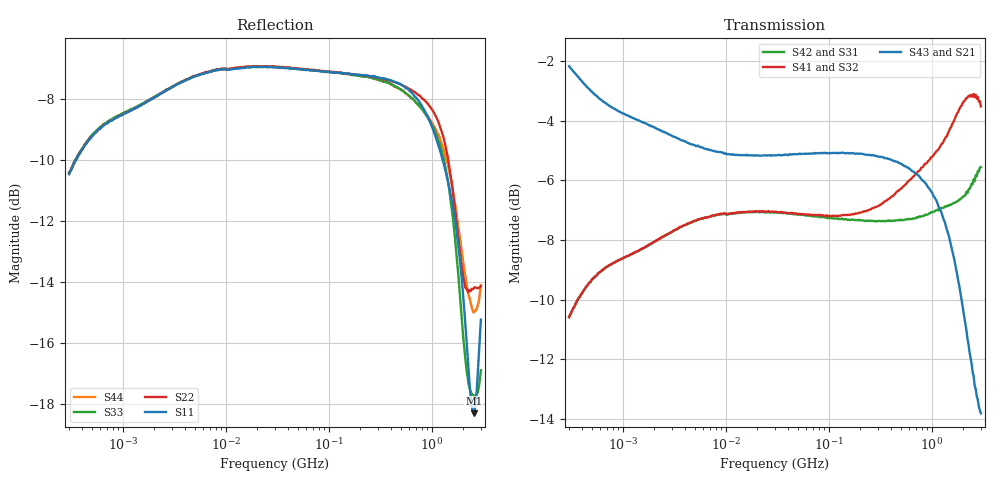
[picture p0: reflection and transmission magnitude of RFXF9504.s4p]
! RFMD Transformer
! RFXF9504 Tested 12/6/2010
! S4P Data File Format
! All S Parameters Mag in dB and Angle in Degree format
! Test Conditions: Input Power = -10dBm @ Temperature +25 deg C
! 401 Frequency points - Log Sweep
! Port 1 is Pin 1,Port 2 is Pin 4, Port 3 is Pin 3 and Port 4 is Pin 2
! FrequencMag(S11)Angle(S1Mag(S12)Angle(S1Mag(S13)Angle(S1Mag(S14)Angle(S14)
!  Mag(S21)Angle(S2Mag(S22)Angle(S2Mag(S23)Angle(S2Mag(S24)Angle(S24)
!  Mag(S31)Angle(S3Mag(S32)Angle(S3Mag(S33)Angle(S3Mag(S34)Angle(S34)
!  Mag(S41)Angle(S4Mag(S42)Angle(S4Mag(S43)Angle(S4Mag(S44)Angle(S44)
# Hz S  dB  R 50
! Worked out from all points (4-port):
!   401 points, 300 kHz to 3 GHz, reference 50 ohm
!   strongest paths, dB at 300 kHz, 3 MHz, 30 MHz, 300 MHz, 3 GHz:
!     S43: -2.2, -4.5, -5.2, -5.2, -13.8
!     S21: -2.2, -4.5, -5.2, -5.2, -14.5
!     S41: -10.6, -7.7, -7.0, -6.9, -3.5
!     S32: -10.6, -7.7, -7.1, -6.9, -3.5
!     S42: -10.6, -7.7, -7.1, -7.4, -5.5
!     S31: -10.6, -7.7, -7.1, -7.4, -5.3
!   lowest |S11| = -18.3 dB at 2.553 GHz (marker M1), VSWR 1.28, Z = 63.3 + j3.69 ohm
!   |S11| at or under -10 dB: start of sweep to 352.5 kHz; 1.274 GHz to end of sweep
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300000  -10.48 36.5  -2.18 -13.2  -10.54 -143.6  -10.54 -143.6
        -2.18 -13.1  -10.46 36.6  -10.53 36.5  -10.54 -143.3
        -10.58 -143.5  -10.56 36.6  -10.42 35.8  -2.17 -13.2
        -10.59 36.7  -10.58 -143.4  -2.17 -13.2  -10.43 36.1
386474.9  -9.76 30.7  -2.63 -12.9  -9.84 -149.3  -9.84 -149.3
          -2.63 -12.9  -9.76 30.8  -9.83 30.7  -9.86 -149.1
          -9.86 -149.2  -9.84 30.8  -9.72 30.2  -2.62 -12.9
          -9.86 30.9  -9.86 -149.2  -2.62 -12.9  -9.74 30.4
433631.9  -9.51 28.2  -2.82 -12.6  -9.59 -151.8  -9.59 -151.8
          -2.81 -12.6  -9.49 28.2  -9.58 28.2  -9.60 -151.7
          -9.60 -151.7  -9.58 28.3  -9.48 27.7  -2.82 -12.6
          -9.60 28.3  -9.59 -151.6  -2.81 -12.5  -9.48 28.0
443732.5  -9.46 27.6  -2.85 -12.6  -9.55 -152.3  -9.55 -152.3
          -2.86 -12.5  -9.45 27.8  -9.53 27.7  -9.55 -152.2
          -9.55 -152.3  -9.54 27.9  -9.42 27.2  -2.85 -12.5
          -9.54 27.8  -9.56 -152.0  -2.86 -12.4  -9.42 27.4
3.444461e8  -7.34 -15.9  -5.29 -16.2  -7.36 156.6  -7.36 156.6
            -5.29 -16.0  -7.37 -15.1  -6.75 5.3  -7.36 158.1
            -7.34 156.7  -6.76 5.3  -7.44 -17.8  -5.23 -15.4
            -6.71 5.8  -7.37 158.1  -5.25 -15.3  -7.44 -15.7
2.553414e9  -18.31 13.7  -12.92 -112.9  -5.69 54.3  -5.69 54.3
            -12.88 -113.2  -14.22 5.2  -3.04 -21.8  -5.98 58.6
            -5.70 53.6  -3.07 -22.2  -17.74 18.9  -12.61 -114.5
            -3.10 -18.4  -5.96 58.4  -12.57 -114.2  -15.01 9.2
3e9  -15.24 21.0  -14.63 -138.7  -5.40 40.1  -5.40 40.1
     -14.53 -138.5  -14.14 -2.6  -3.57 -31.9  -5.65 44.8
     -5.27 40.1  -3.51 -32.4  -16.90 8.9  -13.93 -145.4
     -3.52 -27.8  -5.55 44.6  -13.81 -144.9  -14.11 4.3
